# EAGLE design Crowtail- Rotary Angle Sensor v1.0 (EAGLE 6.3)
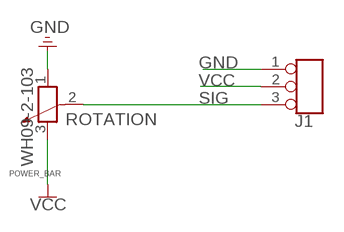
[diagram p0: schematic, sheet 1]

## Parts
J1  TINKER_3P_DIP  [3P_2.0_DIP]
ROTATION  WH09-2-103  R-POTENTIOMETER'WH09-2'  [3P-SQUA-11X9.8X12H]

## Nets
GND: J1.1 ROTATION.1
SIG: J1.3 ROTATION.2
VCC: J1.2 ROTATION.3 ; supply symbol labelled POWER_BAR

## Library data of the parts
J1 = Connector:TINKER_3P_DIP
ROTATION = Discrete:R-POTENTIOMETER*: Potentiometer

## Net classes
0 default: width 0.203 mm, drill 0.305 mm, clearance 0.203 mm

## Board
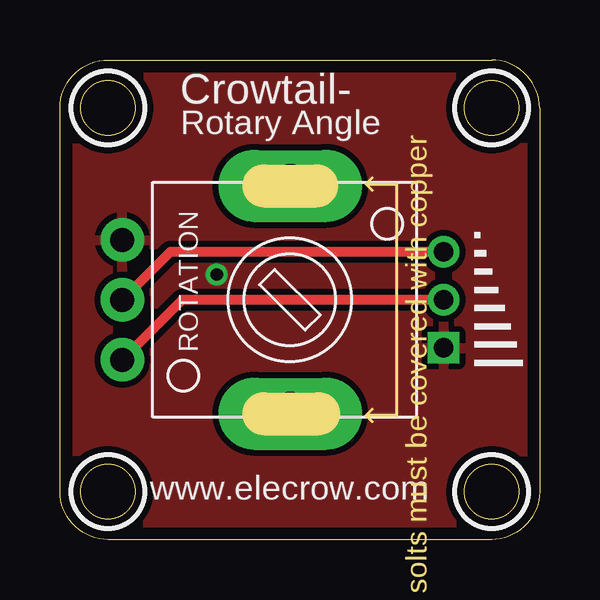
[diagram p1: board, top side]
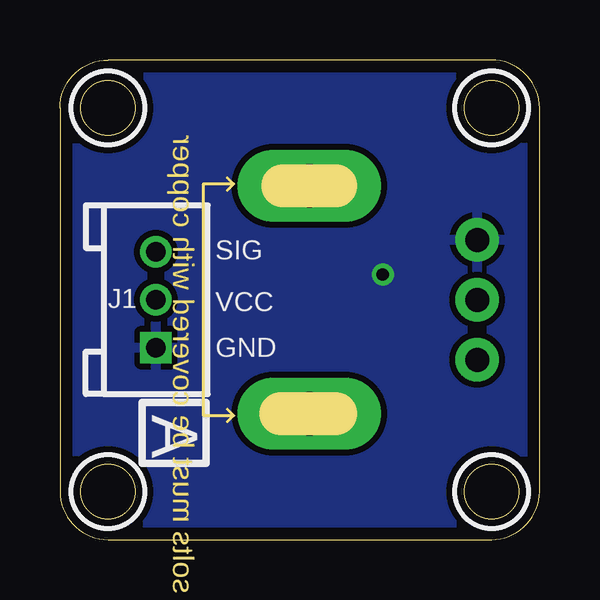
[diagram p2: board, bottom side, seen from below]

Size 20 x 20 mm. Coordinates in mm from the lower left corner, seen from the top.
Outline: 20,18 20,2 arc-90 18,0 2,0 arc-90 0,2 0,18 arc-90 2,20 18,20 arc-90 20,18
Outline: circle at 18,18 radius 1.14
Outline: circle at 18,2 radius 1.14
Outline: circle at 2,18 radius 1.14
Outline: circle at 2,2 radius 1.14
Copper layers (1*16): Top 0.035mm / dielectric 1.5mm / Bottom 0.035mm
Design rules "default *": minimum track width 10mil, minimum drill 20mil, track to track 8mil, track to pad 8mil, pad to pad 8mil, via to via 8mil, smd to smd 8mil, copper to edge 20mil, drill to drill 8mil, minimum pad ring 10mil, minimum via ring 8mil, stop-mask expansion 4mil, vias tented up to drill 100mil, thermal gap 10mil
tRestrict: area 16.5,16.5 to 19.5,19.5; area 16.5,0.5 to 19.5,3.5; area 0.5,16.5 to 3.5,19.5; area 0.5,0.5 to 3.5,3.5
bRestrict: area 16.5,16.5 to 19.5,19.5; area 16.5,0.5 to 19.5,3.5; area 0.5,16.5 to 3.5,19.5; area 0.5,0.5 to 3.5,3.5

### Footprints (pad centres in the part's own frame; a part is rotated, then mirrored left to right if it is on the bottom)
3P_2.0_DIP = drill 0.8 pad 1.27 square: 1 -2,0 | drill 0.8 pad 1.27: 2 0,0; 3 2,0
3P-SQUA-11X9.8X12H = drill 1 pad 1.8: 1 0,2.5; 2 0,0; 3 0,-2.5 | drill 1.8 pad 3 long: P1 7,4.75; P2 7,-4.75

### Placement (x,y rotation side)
J1  16,10 90 bottom
ROTATION  2.6,10 0 top

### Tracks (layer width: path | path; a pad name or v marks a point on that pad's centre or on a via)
GND  (via drill 0.51)
  other vias: 6.54,11.05
  pour Top (isolate 0.254): 20.51,-0.76 -0.45,-0.89 -0.32,20.32 20.64,20.45
  pour Bottom (isolate 0.254): 20.51,-0.89 -0.45,-0.89 -0.32,20.45 20.64,20.45
SIG
  Top 0.406: J1.3 4.6,12 ROTATION.2
VCC
  Top 0.406: J1.2 5.1,10 ROTATION.3

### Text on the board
tPlace: Crowtail- | Rotary Angle | www.elecrow.com
bPlace: SIG | VCC | GND | A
